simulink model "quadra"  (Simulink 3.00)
settings: Solver=ode45  StartTime=0.0  StopTime=5  MaxStep=0.01  RelTol=1e-3  AbsTol=1e-3

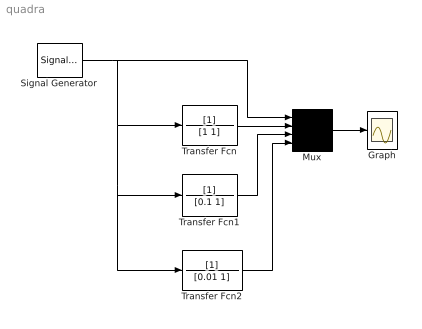
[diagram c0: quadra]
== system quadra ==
  Graph : Scope
  Mux : Mux  Inputs=4
  Signal Generator : SignalGenerator  WaveForm=square  Amplitude=1.000000  Frequency=6.280000  Units=rad/sec
  Transfer Fcn : TransferFcn  Numerator=[1]  Denominator=[1 1]
  Transfer Fcn1 : TransferFcn  Numerator=[1]  Denominator=[0.1 1]
  Transfer Fcn2 : TransferFcn  Numerator=[1]  Denominator=[0.01 1]
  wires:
  Mux/1 -> Graph/1
  Signal Generator/1 -> Mux/1, Transfer Fcn/1, Transfer Fcn1/1, Transfer Fcn2/1
  Transfer Fcn/1 -> Mux/2
  Transfer Fcn1/1 -> Mux/3
  Transfer Fcn2/1 -> Mux/4
